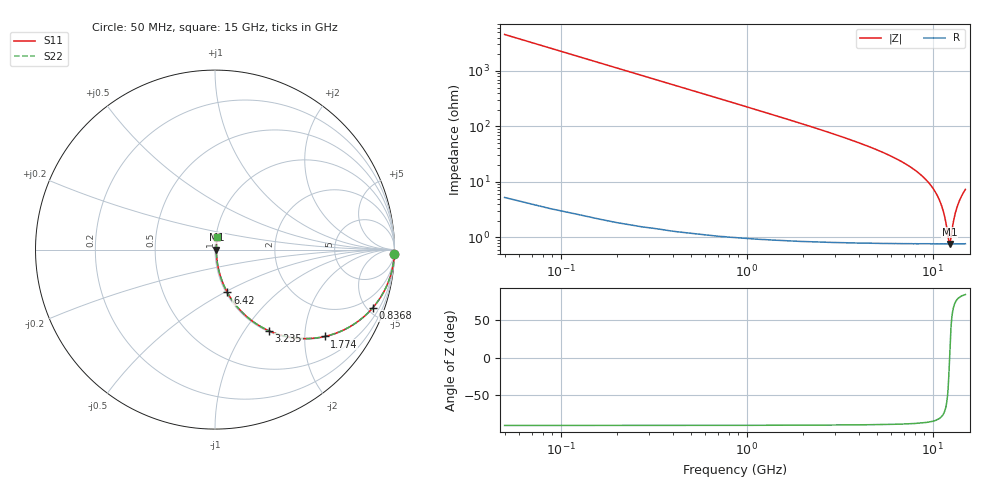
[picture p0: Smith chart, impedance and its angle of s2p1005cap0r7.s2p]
!	AVX	Thin	Film	Operation
!	Date:	March 2012
!	Description: Ultra-Miniature 01005 Size ACCU - P® Thin Film RF / Microwave Capacitor
!	Part Number:  C005YJ0R7ABSTR
!	Serial	Measurements
#	MHz	S	db	R	50
!	S11	S21	S12	S22
!	dB	Phase	dB	Phase	dB	Phase	dB	Phase
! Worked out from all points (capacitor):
!   400 points, 50 MHz to 15 GHz, reference 50 ohm
!   read as one part in series: C = 700 fF near 124.9 MHz
!   lowest |Z| = 764 mohm at 12.34 GHz (marker M1)
!   series resonance near 12.33 GHz, so ESL is about 240 pH
!   S11 on the Smith chart (normalised r, x): 50 MHz: 1, -91; 836.8 MHz: 1.02, -5.41; 1.774 GHz: 1.02, -2.51; 3.235 GHz: 1.02, -1.31; 6.42 GHz: 1.02, -0.52; 15 GHz: 1.02, +0.15
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50  -0.00 -1.3  -33.16 88.7  -33.16 88.7  -0.00 -1.3
87.469  -0.01 -2.2  -28.30 87.7  -28.30 87.7  -0.01 -2.2
124.937  -0.01 -3.1  -25.21 86.8  -25.21 86.8  -0.01 -3.1
274.812  -0.07 -6.9  -18.41 83.0  -18.41 83.0  -0.07 -6.9
499.624  -0.21 -12.4  -13.36 77.4  -13.36 77.4  -0.21 -12.4
836.842  -0.57 -20.3  -9.21 69.5  -9.21 69.5  -0.57 -20.3
1773.559  -2.16 -38.4  -4.14 51.2  -4.14 51.2  -2.16 -38.4
2560.401  -3.82 -49.3  -2.40 40.1  -2.40 40.1  -3.82 -49.3
3234.837  -5.28 -56.3  -1.60 33.0  -1.60 33.0  -5.28 -56.3
5070.802  -9.20 -68.5  -0.62 20.3  -0.62 20.3  -9.20 -68.5
6419.674  -12.10 -73.9  -0.34 14.4  -0.34 14.4  -12.10 -73.9
7543.734  -14.70 -77.1  -0.22 10.6  -0.22 10.6  -14.70 -77.1
10016.67  -22.30 -80.0  -0.09 4.4  -0.09 4.4  -22.30 -80.0
11328.07  -29.91 -74.5  -0.07 1.8  -0.07 1.8  -29.91 -74.5
11702.76  -33.73 -67.3  -0.07 1.1  -0.07 1.1  -33.73 -67.3
12189.85  -41.24 -28.7  -0.07 0.2  -0.07 0.2  -41.24 -28.7
12339.72  -42.40 2.0  -0.07 -0.0  -0.07 -0.0  -42.40 2.0
12527.07  -40.41 37.0  -0.07 -0.3  -0.07 -0.3  -40.41 37.0
12939.22  -34.34 65.7  -0.07 -1.0  -0.07 -1.0  -34.34 65.7
13426.32  -29.87 74.6  -0.07 -1.8  -0.07 -1.8  -29.87 74.6
14100.75  -26.06 78.4  -0.08 -2.8  -0.08 -2.8  -26.06 78.4
15000  -22.81 79.9  -0.09 -4.1  -0.09 -4.1  -22.81 79.9
